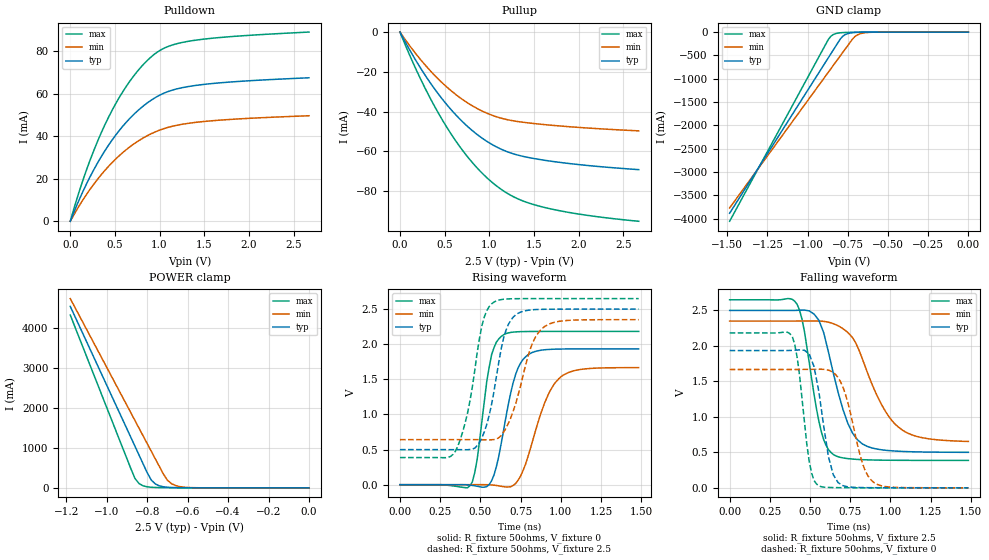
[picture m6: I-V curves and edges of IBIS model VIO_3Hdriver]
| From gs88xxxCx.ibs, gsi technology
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|  signals   DQA1-DQA9, DQB1-DQB9, DQC1-DQC9, DQD1-DQD9
[Model]   VIO_3Hdriver
Model_type   I/O
Polarity   Non-Inverting
Vinl  =   0.8v
Vinh  =   2.0v
Vmeas =   1.5v
Cref  =   0.0pF
Rref  =   50
Vref  =   1.5v
|  variable   typ   min   max
C_comp   3.0pF   2.5pF   3.5pF
|  variable   typ   min   max
[Temperature Range]   50   0   100
|  variable   typ   min   max
[Voltage Range]   2.5   2.35   2.65
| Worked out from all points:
|   slope of the pulldown table from 0 to 0.375 V, typ, clamps not added: 11.6 ohm
|   slope of the pullup table from 0 to 0.375 V, typ, clamps not added: 13.5 ohm
|   GND clamp passes 1 mA (typ) near -0.61 V on its own axis
|   POWER clamp passes 1 mA (typ) near -0.59 V on its own axis
|   rising waveform, R_fixture 50ohms, V_fixture 0: 20-80 % time 104ps typ, 146ps min, 76.6ps max; typ from 0 V to 1.93 V
|   rising waveform, R_fixture 50ohms, V_fixture 2.5: 20-80 % time 101ps typ, 129ps min, 104ps max; typ from 0.5 V to 2.5 V
|   falling waveform, R_fixture 50ohms, V_fixture 2.5: 20-80 % time 143ps typ, 204ps min, 99.6ps max; typ from 2.5 V to 0.5 V
|   falling waveform, R_fixture 50ohms, V_fixture 0: 20-80 % time 82ps typ, 110ps min, 65.5ps max; typ from 1.93 V to 0 V
[Pulldown]
| voltage   typ   min   max
0V        -354.4pA   -1.034nA   -211.5pA
108mV     10.89mA    7.806mA    15.02mA
216mV     20.44mA    14.69mA    28.09mA
324mV     28.77mA    20.73mA    39.42mA
432mV     36mA       25.98mA    49.21mA
540mV     42.23mA    30.51mA    57.61mA
675mV     48.74mA    35.24mA    66.36mA
810mV     53.96mA    39.02mA    73.36mA
945mV     57.99mA    41.92mA    78.67mA
1.134V    61.57mA    44.6mA     82.79mA
1.404V    63.89mA    46.52mA    85.18mA
2.673V    67.5mA     49.63mA    89.01mA
[Pullup]
| voltage (VDDQ-Vout)   typ   min   max
0V        266.7pA    1.042nA    119pA
243mV     -19.01mA   -14.52mA   -24.74mA
378mV     -27.99mA   -21.3mA    -36.57mA
513mV     -35.9mA    -27.19mA   -47.06mA
648mV     -42.73mA   -32.2mA    -56.26mA
783mV     -48.53mA   -36.37mA   -64.19mA
918mV     -53.32mA   -39.7mA    -70.9mA
1.053V    -57.13mA   -42.21mA   -76.41mA
1.296V    -61.61mA   -44.86mA   -83.41mA
1.566V    -64.13mA   -46.34mA   -87.65mA
2.025V    -66.79mA   -48.05mA   -91.73mA
2.673V    -69.22mA   -49.72mA   -95.2mA
[GND Clamp]
| voltage   typ   min   max
-1.485V   -3.884A    -3.771A    -4.056A
-885mV    -626.9mA   -926.9mA   -247.2mA
-870mV    -545.6mA   -856mA     -153.5mA
-855mV    -464.4mA   -785mA     -89.11mA
-825mV    -301.9mA   -643.2mA   -32.88mA
-795mV    -141.5mA   -501.4mA   -15.38mA
-780mV    -86.61mA   -430.5mA   -11.65mA
-750mV    -32.85mA   -288.8mA   -7.734mA
-705mV    -8.727mA   -95.28mA   -4.834mA
-660mV    -2.907mA   -24.97mA   -2.925mA
-555mV    -316.7uA   -1.176mA   -484.9uA
0V        -354.4pA   -1.034nA   -211.5pA
[POWER Clamp]
| voltage (VDDQ-Vout)   typ   min   max
-1.18V    4.545A     4.74A      4.328A
-880mV    1.258A     1.875A     474.1mA
-860mV    1.039A     1.684A     234.3mA
-840mV    820.4mA    1.493A     107.4mA
-820mV    601.5mA    1.302A     50.64mA
-780mV    197.3mA    920.5mA    14.28mA
-760mV    99.71mA    729.7mA    9.034mA
-720mV    26.23mA    348.2mA    4.898mA
-700mV    13.96mA    192.6mA    3.916mA
-660mV    4.495mA    57.55mA    2.579mA
-560mV    510.5uA    2.941mA    648.3uA
0V        285pA      1.042nA    119.1pA
[Ramp]
| voltage   typ   min   max
dV/dt_r   1.60/124p   1.42/174p   1.84/96p
dV/dt_f   1.62/126p   1.44/176p   1.85/96p
R_load  =   50ohms
[Rising Waveform]
C_fixture =   0.0pF
R_fixture =   50ohms
V_fixture =   0
| Time   V(typ)   V(min)   V(max)
0s        2.78nV     10.68nV    1.252nV
435ps     -5.969mV   384.7uV    -14.98mV
480ps     -22.23mV   527.1uV    356mV
570ps     55.14mV    -3.64mV    1.85V
645ps     777.5mV    -27.7mV    2.135V
720ps     1.573V     16.62mV    2.176V
795ps     1.848V     390mV      2.182V
900ps     1.921V     1.165V     2.183V
1.005ns   1.932V     1.544V     2.183V
1.485ns   1.934V     1.667V     2.183V
[Rising Waveform]
C_fixture =   0.0pF
R_fixture =   50ohms
V_fixture =   2.5
V_fixture_min =  2.35
V_fixture_max =  2.65
| Time   V(typ)   V(min)   V(max)
0s        499.5mV    641.7mV    386.6mV
345ps     498.8mV    641.7mV    477mV
420ps     497.8mV    642mV      1.015V
495ps     602.1mV    641.1mV    2.087V
540ps     859mV      639.1mV    2.477V
585ps     1.328V     642.2mV    2.601V
675ps     2.286V     876.7mV    2.646V
810ps     2.488V     1.929V     2.65V
885ps     2.497V     2.224V     2.65V
1.485ns   2.5V       2.35V      2.65V
[Falling Waveform]
C_fixture =   0.0pF
R_fixture =   50ohms
V_fixture =   2.5
V_fixture_min =  2.35
V_fixture_max =  2.65
| Time   V(typ)   V(min)   V(max)
0s        2.5V       2.35V      2.65V
420ps     2.501V     2.35V      2.585V
465ps     2.505V     2.351V     2.208V
555ps     2.362V     2.35V      940.1mV
645ps     1.615V     2.313V     469.6mV
735ps     909.9mV    2.189V     411.9mV
825ps     620mV      1.82V      397mV
945ps     535.9mV    1.173V     390mV
1.05ns    515.7mV    855.2mV    387.9mV
1.485ns   500.5mV    653.4mV    386.6mV
[Falling Waveform]
C_fixture =   0.0pF
R_fixture =   50ohms
V_fixture =   0
| Time   V(typ)   V(min)   V(max)
0s        1.934V     1.667V     2.183V
390ps     1.937V     1.667V     2.131V
420ps     1.941V     1.668V     1.839V
495ps     1.887V     1.67V      371.3mV
555ps     1.355V     1.671V     26.94mV
615ps     435.4mV    1.658V     5.299mV
675ps     73.29mV    1.554V     2.572mV
825ps     3.537mV    354.2mV    637.1uV
885ps     2.101mV    98.74mV    359.5uV
1.485ns   27.17uV    301.2uV    2.067uV
